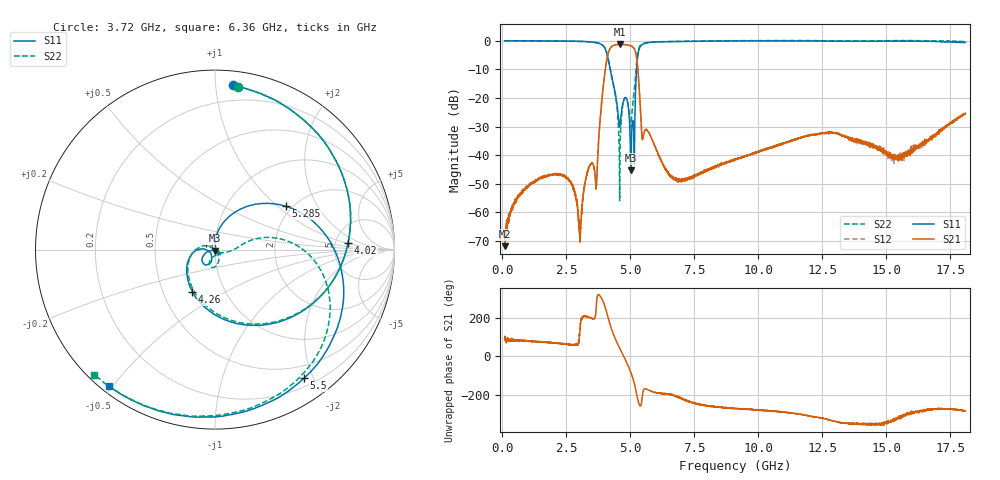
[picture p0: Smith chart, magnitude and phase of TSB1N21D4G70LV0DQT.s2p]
! TSB1N21D4G70LV0DQT  S-PARAMETER MODEL  ( General Type )
! Model Generated by TAIYO YUDEN Corporation (https://www.yuden.co.jp/en/)
! Version 1.0
! TAIYO YUDEN Control No. 20240527
! Copyright(c) 2024 TAIYO YUDEN CO.,LTD. All Rights Reserved.
! Products Name : Ceramic RF Devices
! Characteristics :
!  Passband freq : 4400-5000MHz ( At Passband , Insertion Loss : 2.5dB , VSWR 2.0 )
!  Attenuation : 35 dB min at 100 to 3600MHz, 15 dB min at 5490 to 5925MHz, Impedance : 50 Ohm
!  Case Size : 2 x 1.25 / 0.079 x 0.049 [mm/inch] , Thickness : 0.65/ 0.026 [mm/inch]
!  (Conditions: Temperature = 25 degC , DC Bias Current/Voltage = 0A / 0V)
! External Node Assignments :
!  1  o---|-------|---o  2
!  |  BPF  |
! GND o---|-------|---o GND
! Frequency Range : 100MHz  -  18.1GHz  [ 3601 STEP ]
# MHZ S RI R 50
! Freq[MHz].  S11 Real  S11 Imag  S21 Real  S21 Imag  S12 Real  S12 Imag  S22 Real  S22 Imag
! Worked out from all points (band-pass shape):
!   3601 points, 100 MHz to 18.1 GHz, reference 50 ohm
!   highest |S21| = -1.24 dB at 4.61 GHz (marker M1); lowest = -71.8 dB at 110 MHz (marker M2)
!   |S21| within 3 dB of the highest: 4.15 GHz to 5.224 GHz (1.075 GHz wide, 22.9 % of centre)
!   lowest |S11| = -45.3 dB at 5.03 GHz (marker M3), VSWR 1.01, Z = 50 - j0.545 ohm
!   |S11| at or under -10 dB: 4.227 GHz to 5.256 GHz (1.029 GHz wide, 21.7 % of centre)
!   |S22| runs from -55.9 to 0.1 dB; largest |S21 - S12| = 0.0044
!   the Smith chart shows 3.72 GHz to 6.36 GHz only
!   S11 on the Smith chart (normalised r, x): 3.72 GHz: 0.09, +1.11; 4.02 GHz: 6.58, +1.05; 4.26 GHz: 0.70, -0.36; 5.285 GHz: 1.86, +1.14; 5.5 GHz: 0.31, -1.87; 6.36 GHz: 0.02, -0.49
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100  -1.001 0.0194  -1.63e-05 0.000422  -2.99e-05 0.000257  -0.9982 0.02
110  -1.001 0.0212  -5.76e-05 0.00025  0.000104 0.000368  -0.9984 0.0211
1715  -0.9534 0.2841  0.00132 0.00418  0.00138 0.00395  -0.9451 0.2914
2610  -0.8515 0.4999  0.00169 0.0032  0.00193 0.0032  -0.8363 0.516
3100  -0.6843 0.6984  -0.000898 -0.000298  -0.000825 -0.000289  -0.6605 0.7151
3350  -0.4995 0.8263  -0.00486 -0.00221  -0.00488 -0.00227  -0.4703 0.8379
3720  0.1005 0.9148  0.00415 -0.00475  0.00424 -0.00475  0.1291 0.9082
4020  0.7412 0.0358  -0.0586 -0.2807  -0.0588 -0.2806  0.7422 0.0369
4260  -0.126 -0.2351  -0.6506 0.4181  -0.6514 0.4184  -0.1123 -0.2414
4425  -0.1181 -0.013  0.00152 0.8479  0.00129 0.8484  -0.1148 -0.00642
4610  -0.0204 -0.0273  0.6928 0.5209  0.6919 0.5208  0.00824 -0.0097
4790  -0.0518 -0.0856  0.8389 -0.1724  0.839 -0.172  -0.00314 -0.0978
5030  -4.49e-05 -0.00545  0.0787 -0.8133  0.0788 -0.8133  0.017 -0.0253
5105  0.0309 -0.0258  -0.3097 -0.716  -0.3091 -0.7162  0.0753 -0.0116
5285  0.3962 0.2409  -0.3226 0.2311  -0.3225 0.2313  0.5452 -0.0515
5500  0.4958 -0.7174  -0.0192 0.00333  -0.0195 0.00326  0.2944 -0.839
6100  -0.4188 -0.8587  -0.0101 0.00208  -0.0103 0.00222  -0.524 -0.8042
6360  -0.5909 -0.7614  -0.00568 0.00144  -0.00566 0.00148  -0.6718 -0.6965
9100  -0.9945 -0.0321  0.000482 0.00846  0.000601 0.00854  -1.005 0.0271
12100  -0.9647 0.2513  0.0158 0.0163  0.0158 0.0164  -0.9666 0.2809
15100  -0.9841 -0.0759  0.0103 0.00278  0.0113 0.00301  -1.004 -0.0315
18100  -0.9271 0.1424  0.013 0.0518  0.0152 0.0512  -0.9417 0.1967
